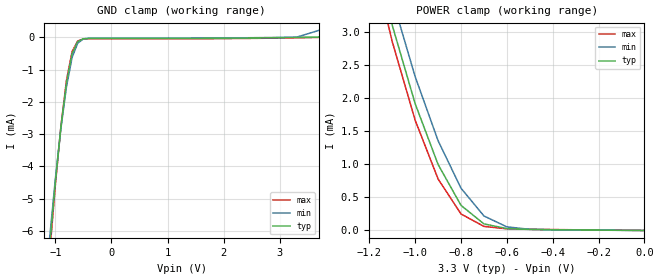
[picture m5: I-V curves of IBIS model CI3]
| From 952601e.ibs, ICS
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|   Model CI3
[Model]   CI3
Model_type   Input
Polarity   Inverting
Vinl =   0.80V
Vinh =   2.00V
C_comp   5.50pF   5.00pF   6.00pF
[Temperature Range]   27.00   70.00   0.000
[Voltage Range]   3.30V   3.00V   3.70V
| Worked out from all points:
|   GND clamp passes 1 mA (typ) near -0.75 V on its own axis
|   POWER clamp passes 1 mA (typ) near -0.90 V on its own axis
[GND_clamp]
| voltage   I(typ)   I(min)   I(max)
-3.3V     -62.1mA    -58.1mA    -64.96mA
-1.1V     -6.5mA     -6.22mA    -6.72mA
-1V       -4.52mA    -4.42mA    -4.61mA
-900mV    -2.79mA    -2.83mA    -2.77mA
-800mV    -1.41mA    -1.53mA    -1.33mA
-700mV    -500uA     -620uA     -440uA
-600mV    -130uA     -180uA     -110uA
-500mV    -42.15uA   -47.42uA   -49.41uA
-400mV    -31.3uA    -25.2uA    -43.22uA
3.3V      64.28pA    7.06uA     -12.09uA
3.7V      11.66uA    220uA      7.53nA
[POWER_clamp]
| voltage   I(typ)   I(min)   I(max)
-3.3V     65.46mA    62.39mA    68.37mA
-1.2V     4.51mA     4.87mA     4.31mA
-1.1V     3.11mA     3.51mA     2.86mA
-1V       1.92mA     2.33mA     1.67mA
-900mV    1mA        1.36mA     780uA
-800mV    380uA      640uA      250uA
-700mV    100uA      220uA      61.82uA
-600mV    28.45uA    54.53uA    25.09uA
-500mV    15.73uA    17.8uA     17.86uA
0V        64.28pA    2.84nA     7.53nA
